FUNCTION F_TwoPoints : LREAL	// 使用直线上的两个点
VAR_INPUT
    x1, y1: 		LREAL;	// 直线上的点A坐标
    x2, y2: 		LREAL;	// 直线上的点B坐标
    x0, y0: 		LREAL;	// 点P坐标
END_VAR
VAR
    crossProduct: 	LREAL;	//向量积
    abLength: 		LREAL;	//AB向量的长度
    dx, dy: 		LREAL;
END_VAR

// 计算向量分量
dx := x2 - x1;
dy := y2 - y1;

// 计算叉乘的绝对值：(x2-x1)*(y0-y1) - (y2-y1)*(x0-x1)
CrossProduct := ABS(dx * (y0 - y1) - dy * (x0 - x1));

// 计算AB向量的长度
abLength := SQRT(dx * dx + dy * dy);

// 避免除零错误
IF abLength = 0 THEN
	F_TwoPoints := 0.0;
ELSE
    F_TwoPoints := CrossProduct / abLength;
END_IF;

END_FUNCTION
